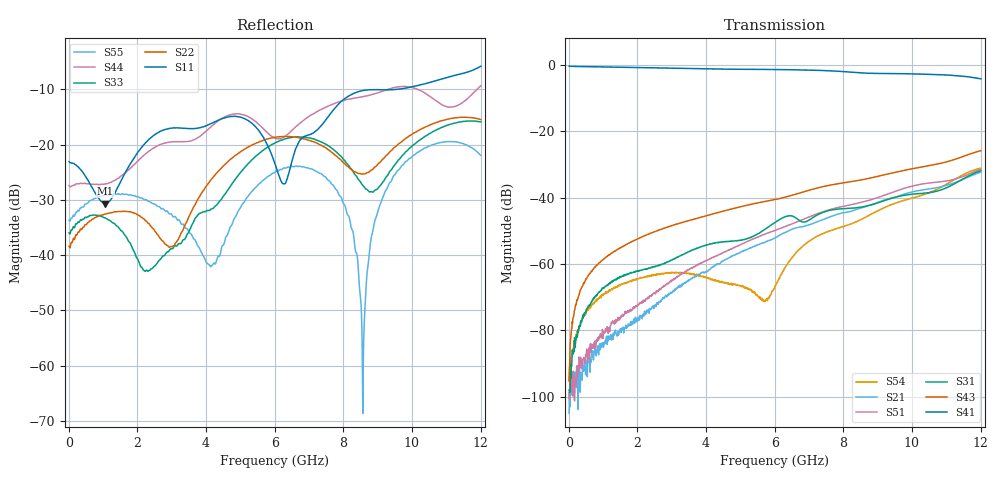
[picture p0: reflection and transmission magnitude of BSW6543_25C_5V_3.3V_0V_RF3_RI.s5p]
! Agilent Technologies	N5230C	MY49001333	A.09.33.09
!	Test time	=	2026-05-28 10:00
!	Product	=	BSW6543
!	Temp	=	25C
!	Logic	=	RF3
!	Port1	=	RFC
!	Port2	=	RF1
!	Port3	=	RF2
!	Port4	=	RF3
!	Port5	=	RF4
!S5P File: Measurements: <S11,S12,S13,S14,S15>,
!<S21,S22,S23,S24,S25>,
!<S31,S32,S33,S34,S35>,
!<S41,S42,S43,S44,S45>,
!<S51,S52,S53,S54,S55>;
# HZ S RI R 50
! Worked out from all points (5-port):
!   1201 points, 10 MHz to 12.01 GHz, reference 50 ohm
!   strongest paths, dB at 10 MHz, 3.01 GHz, 6.01 GHz, 9.01 GHz, 12.01 GHz:
!     S41: -0.4, -1.1, -1.5, -2.6, -4.3
!     S43: -95.3, -48.5, -40.6, -33.6, -25.9
!     S31: -98.0, -58.8, -47.5, -41.6, -31.9
!     S51: -98.8, -64.8, -49.9, -40.0, -31.4
!     S21: -105.0, -68.6, -52.2, -41.5, -32.4
!     S54: -95.0, -62.7, -66.7, -44.0, -31.1
!   lowest |S11| = -30.7 dB at 1.07 GHz (marker M1), VSWR 1.06, Z = 47.2 - j0.566 ohm
!   |S11| at or under -10 dB: start of sweep to 9.565 GHz
